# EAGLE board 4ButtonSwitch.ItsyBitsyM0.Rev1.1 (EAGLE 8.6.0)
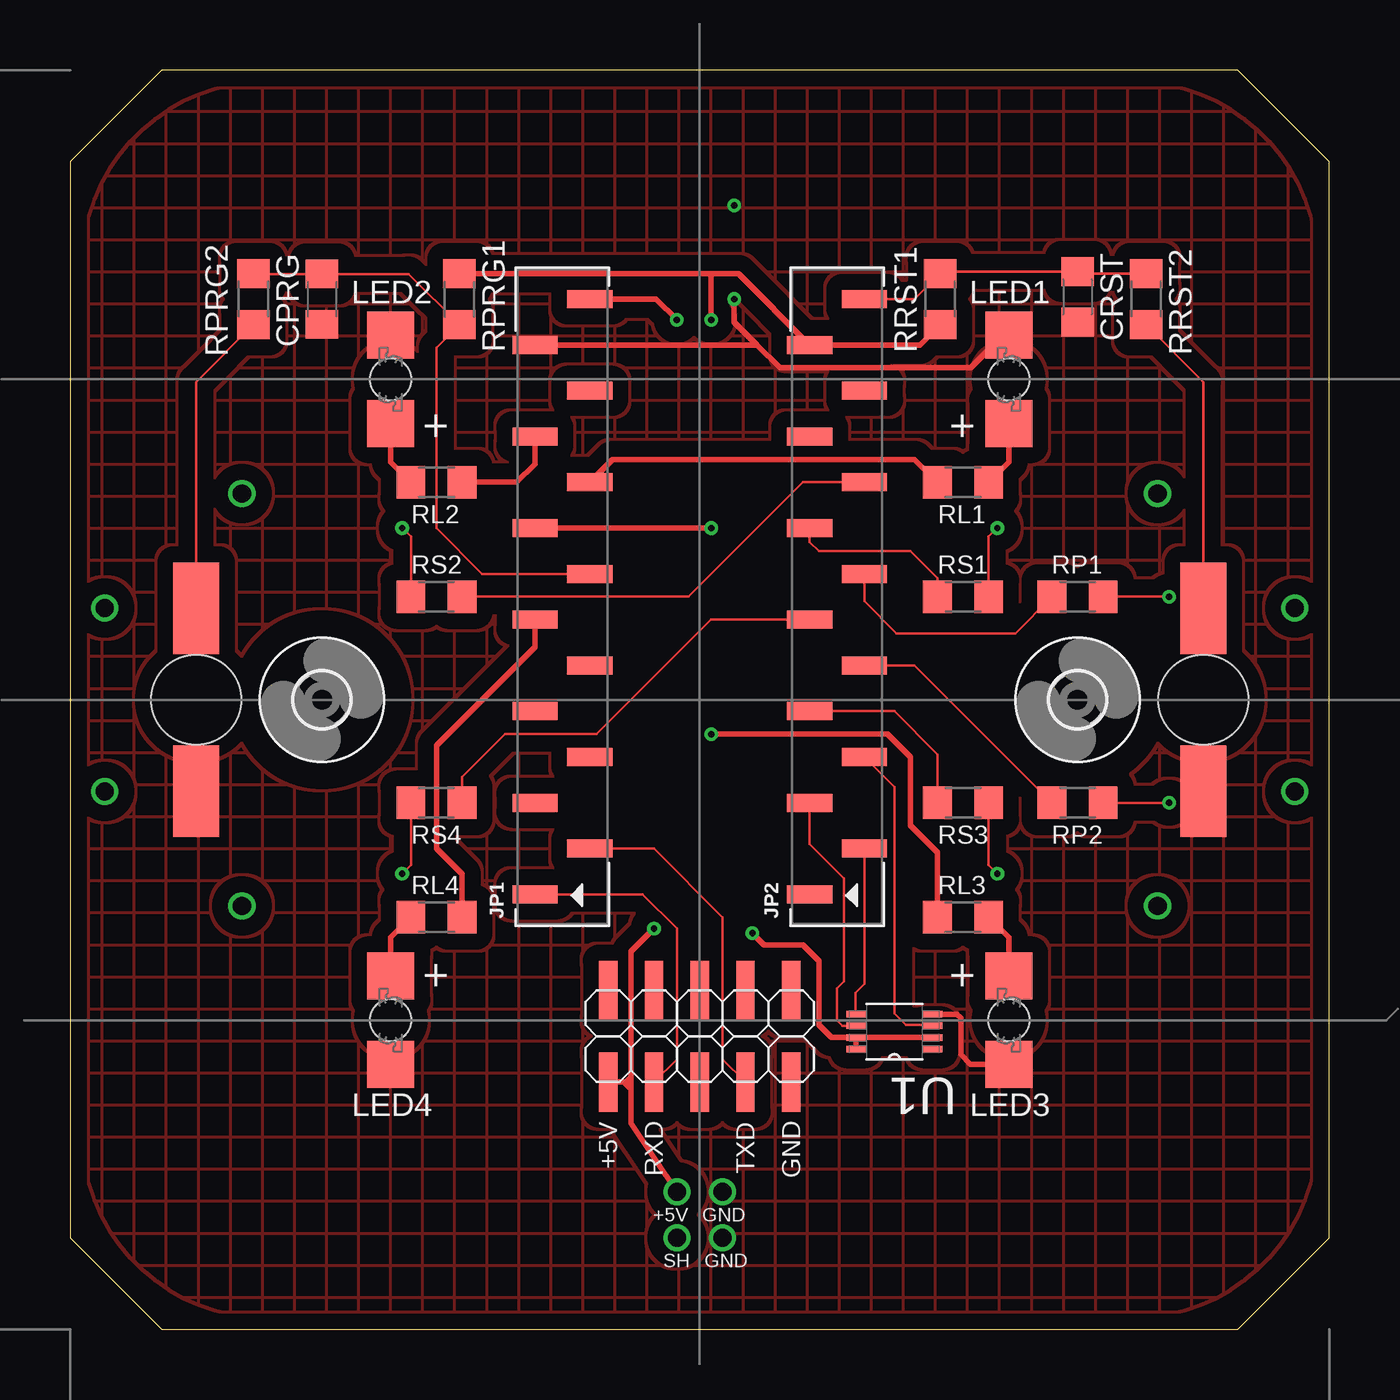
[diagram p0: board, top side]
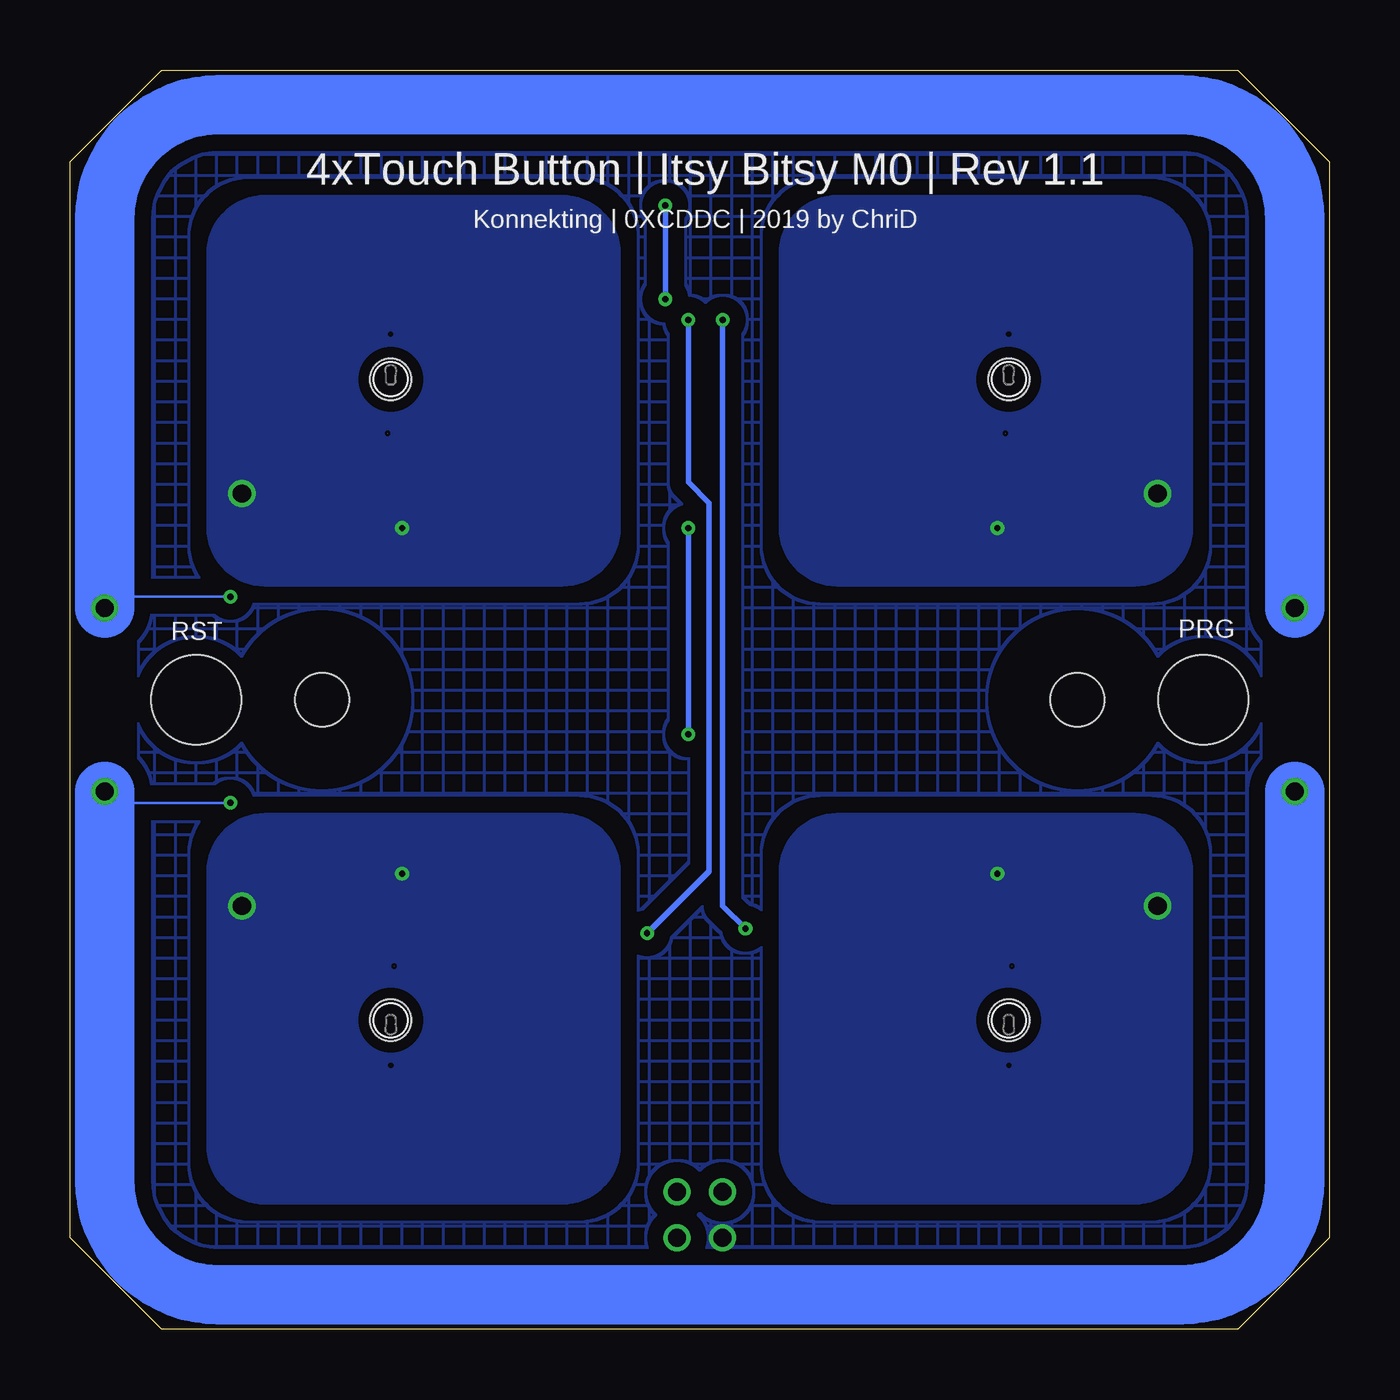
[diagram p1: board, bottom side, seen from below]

Size 69.85 x 69.85 mm. Coordinates in mm from the lower left corner, seen from the top.
Outline: 5.08,69.85 64.77,69.85 69.85,64.77 69.85,5.08 64.77,0 5.08,0 0,5.08 0,64.77 5.08,69.85
Outline: 6.34,69.84 5.08,69.85
Copper layers (1*16): Top 0.035mm / dielectric 1.5mm / Bottom 0.035mm
Design rules "konnektduino": minimum track width 6mil, minimum drill 0.35mm, track to track 6mil, track to pad 6mil, pad to pad 6mil, via to via 6mil, smd to smd 6mil, copper to edge 25mil, drill to drill 6mil, minimum pad ring 10mil, minimum via ring 8mil, stop-mask expansion 1mil, vias tented up to drill 25mil, thermal gap 10mil
Holes 5 mm at 62.87,34.92 6.99,34.92

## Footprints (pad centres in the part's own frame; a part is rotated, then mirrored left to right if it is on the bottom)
C1206 = smd 1.6 x 1.8: 1 -1.4,0; 2 1.4,0
SMD2,54-5,08 = smd 2.54 x 5.08: 1 0,0
1X14_SMT = smd 1 x 2.5: 1 -16.51,1.52; 2 -13.97,-1.52; 3 -11.43,1.52; 4 -8.89,-1.52; 5 -6.35,1.52; 6 -3.81,-1.52; 7 -1.27,1.52; 8 1.27,-1.52; 9 3.81,1.52; 10 6.35,-1.52; 11 8.89,1.52; 12 11.43,-1.52; 13 13.97,1.52; 14 16.51,-1.52
P47F-BOTTOM = smd 2.6 x 2.6: A -2.45,0; C 2.45,0 | hole 2.3: 0,0
R1206 = smd 1.6 x 1.803: 1 -1.422,0; 2 1.422,0
2X05SMD = smd 1.016 x 3.302: 1 -1.27,-3.81; 2 -1.27,1.27; 3 1.27,-3.81; 4 1.27,1.27; 5 3.81,-3.81; 6 3.81,1.27; 7 6.35,-3.81; 8 6.35,1.27; 9 8.89,-3.81; 10 8.89,1.27
SOP65P490X110-8N = smd 1.067 x 0.356: 1 -2.134,0.965; 2 -2.134,0.33; 3 -2.134,-0.33; 4 -2.134,-0.965; 5 2.134,-0.965; 6 2.134,-0.33; 7 2.134,0.33; 8 2.134,0.965
3,0 = hole 3: 0,0

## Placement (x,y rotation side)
CPRG  100nF  [C1206]  13.97,57.15 270 top
CRST  100nF  [C1206]  55.88,57.28 270 top
GND_NRST  0  [SMD2,54-5,08]  6.99,29.84 0 top
GND_PRG  0  [SMD2,54-5,08]  62.87,29.84 0 top
JP1  [1X14_SMT]  27.3,40.64 90 top
JP2  [1X14_SMT]  42.55,40.64 90 top
LED1  LWP4-BOTTOM  [P47F-BOTTOM]  52.07,52.7 90 top
LED2  LWP4-BOTTOM  [P47F-BOTTOM]  17.78,52.7 90 top
LED3  LWP4-BOTTOM  [P47F-BOTTOM]  52.07,17.14 270 top
LED4  LWP4-BOTTOM  [P47F-BOTTOM]  17.78,17.14 270 top
PAD_NRST  0  [SMD2,54-5,08]  62.87,40.01 0 top
PAD_PRG  0  [SMD2,54-5,08]  6.99,40.01 0 top
RL1  330E  [R1206]  49.53,46.99 0 top
RL2  330E  [R1206]  20.32,46.99 180 top
RL3  330E  [R1206]  49.53,22.86 0 top
RL4  330E  [R1206]  20.32,22.86 180 top
RP1  1k  [R1206]  55.88,40.64 180 top
RP2  1k  [R1206]  55.88,29.21 180 top
RPRG1  10k  [R1206]  21.59,57.15 90 top
RPRG2  330E  [R1206]  10.16,57.15 270 top
RRST1  10k  [R1206]  48.26,57.15 270 top
RRST2  330E  [R1206]  59.69,57.15 270 top
RS1  1k  [R1206]  49.53,40.64 180 top
RS2  1k  [R1206]  20.32,40.64 0 top
RS3  1k  [R1206]  49.53,29.21 180 top
RS4  1k  [R1206]  20.32,29.21 0 top
SAM12235-ND  SIEMENS BCU  [2X05SMD]  31.11,17.53 0 top
U1  MAX31723MUA+T  [SOP65P490X110-8N]  45.72,16.51 180 top
U$1  [3,0]  13.97,34.92 0 top
U$2  [3,0]  55.88,34.92 0 top

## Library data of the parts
CPRG CRST = rcl; SPICEPREFIX: C
GND_NRST GND_PRG PAD_NRST PAD_PRG = wirepad
JP1 JP2 = pinhead+
LED1-LED4 = led
RL1-RL4 RP1 RP2 RPRG1 RPRG2 RRST1 RRST2 RS1-RS4 = resistor
SAM12235-ND = pinhead
U1 = MAX31723MUA_T (1); AVAILABILITY: Unavailable; DESCRIPTION: Thermostat Â±2Â°C Digital SMD 8-Pin uMAX T/R; MF: Maxim Integrated; MP: MAX31723MUA+T; PACKAGE: MSOP-8 Maxim Integrated; PRICE: None
U$1 U$2 = holes

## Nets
+3V3: JP2.13 RPRG1.2 RRST1.2 U1.2 U1.7 U1.8
+5V: JP1.14 SAM12235-ND.1
A0: JP2.10 RS2.2
A1: JP2.9 RS1.2
A2: JP2.8 RP1.2
A3: JP2.7 RS4.2
A4: JP2.6 RP2.2
A5: JP2.5 RS3.2
D7: JP1.6
D9: JP1.7 RL4.1
D10: CPRG.1 JP1.8 RPRG1.1 RPRG2.1
D11: JP1.9 RL3.1
D12: JP1.10 RL1.1
D13: JP1.11 RL2.1
GND: CPRG.2 CRST.2 GND_NRST.1 GND_PRG.1 JP1.13 LED1.C LED2.C LED3.C LED4.C SAM12235-ND.9 U1.4
MISO: JP2.2 U1.5
MOSI: JP2.3 U1.6
N$19: LED1.A RL1.2
N$20: LED2.A RL2.2
N$21: LED3.A RL3.2
N$22: LED4.A RL4.2
PRG: PAD_PRG.1 RPRG2.2
RESET: PAD_NRST.1 RRST2.2
RST: CRST.1 JP2.14 RRST1.1 RRST2.1
SCK: JP2.4 U1.3
SCL: JP1.4
SDA: JP1.3
SENS_1: RS1.1
SENS_2: RS2.1
SENS_3: RS3.1
SENS_4: RS4.1
SENS_PROX_1: RP1.1
SENS_PROX_2: RP2.1
USART1_RX: JP1.1 SAM12235-ND.3
USART1_TX: JP1.2 SAM12235-ND.7

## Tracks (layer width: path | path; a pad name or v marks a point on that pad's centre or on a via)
+3V3  (via drill 0.35)
  Top 0.305: 35.56,58.57 37.06,58.57 JP2.13 47.14,54.61 RRST1.2 | 35.56,58.57 RPRG1.2 | U1.8 U1.7 | U1.7 U1.2 | 35.56,58.57 v35.56,56.01 | v37.85,21.97 38.48,21.34 40.64,21.34 41.53,20.45 41.53,16.89 42.24,16.18 U1.7
  Bottom 0.305: v35.56,56.01 35.56,46.99 34.42,45.85 34.42,25.4 v37.85,21.97
+5V  (via drill 0.35, 1)
  Top 0.305: SAM12235-ND.1 30.73,13.72 | 30.73,13.72 30.86,13.72 31.11,13.97 | JP1.14 32.51,57.15 v33.66,56.01 | v33.66,7.62 31.11,11.43 31.11,13.34 | 31.11,13.34 31.11,13.97 | 30.73,13.72 31.11,13.34 | 31.11,13.97 31.11,20.95 v32.38,22.23
  Bottom 0.305: v32.38,22.23 33.66,23.5 v33.66,56.01
A0
  Top 0.152: RS2.2 34.29,40.64 40.64,46.99 JP2.10
A1
  Top 0.152: JP2.9 41.02,43.68 41.53,43.18 46.61,43.18 48.11,41.68 RS1.2
A2
  Top 0.152: JP2.8 44.06,40.39 45.85,38.61 52.43,38.61 RP1.2
A3
  Top 0.152: RS4.2 21.74,30.63 24.13,33.02 29.21,33.02 35.56,39.37 JP2.7
A4
  Top 0.152: JP2.6 46.84,36.83 RP2.2
A5
  Top 0.152: RS3.2 48.11,31.9 45.72,34.29 JP2.5
D9
  Top 0.305: RL4.1 21.74,25.25 20.32,26.67 20.32,32.38 25.79,37.85 JP1.7
D10
  Top 0.152: RPRG2.1 10.18,58.55 CPRG.1 18.77,58.55 RPRG1.1 20.32,54.46 20.32,44.45 22.86,41.91 JP1.8
D11  (via drill 0.35)
  Top 0.305: v35.56,44.45 JP1.9 | v35.56,33.02 45.34,33.02 46.61,31.75 46.61,27.94 48.11,26.44 RL3.1
  Bottom 0.305: v35.56,44.45 v35.56,33.02
D12
  Top 0.305: RL1.1 46.84,48.26 30.09,48.26 JP1.10
D13
  Top 0.305: JP1.11 25.79,48.01 24.77,46.99 RL2.1
GND  (via drill 0.35, 1)
  Top 0.305: 38.1,54.61 39.37,53.34 49.97,53.34 51.27,54.64 51.56,54.64 LED1.C | JP1.13 38.1,54.61 | U1.4 49.2,17.48 49.4,17.27 49.4,15.24 49.95,14.7 LED3.C | 38.1,54.61 36.83,55.88 v36.83,57.15
  Bottom 0.305: v36.83,57.15 v36.83,62.36
  other vias: 36.2,7.62 36.2,5.08
  pour Top (isolate 0.889, rank 6, no thermals, hatched): 0.64,10.79 arc90 10.79,0.64 59.05,0.64 arc90 69.22,10.79 69.22,59.05 arc90 59.05,69.22 10.79,69.22 arc90 0.64,59.05
MISO
  Top 0.152: JP2.2 44.06,19.17 43.56,18.67 43.56,17.5 U1.5
MOSI
  Top 0.152: JP2.3 41.02,26.92 42.93,25.02 42.93,19.3 42.55,18.92 42.55,17.14 42.85,16.84 U1.6
N$19
  Top 0.305: LED1.A 52.07,48.11 RL1.2
N$20
  Top 0.305: LED2.A 17.78,48.11 RL2.2
N$21
  Top 0.305: LED3.A 52.07,21.74 RL3.2
N$22
  Top 0.305: LED4.A 17.78,21.74 RL4.2
PRG
  Top 0.152: PAD_PRG.1 6.99,52.55 RPRG2.2
RESET
  Top 0.152: PAD_NRST.1 62.87,52.55 RRST2.2
RST
  Top 0.152: RRST2.1 55.99,58.57 CRST.1 48.37,58.68 RRST1.1 46.84,57.15 JP2.14
SCK
  Top 0.152: JP2.4 45.72,30.09 45.72,17.53 46.35,16.89 47.8,16.89 U1.3
SENS_1  (via drill 0.35, 1)
  Top 0.152: RS1.1 50.95,43.97 v51.44,44.45
  other vias: 60.33,46.35
  pour Bottom: 39.37,59.69 39.37,44.45 arc90 42.55,41.27 59.05,41.27 arc90 62.23,44.45 62.23,59.69 arc90 59.05,62.87 42.55,62.87 arc90
SENS_2  (via drill 0.35, 1)
  Top 0.152: RS2.1 18.9,43.97 v18.41,44.45
  other vias: 9.53,46.35
  pour Bottom: 10.79,41.27 27.3,41.27 arc90 30.48,44.45 30.48,59.69 arc90 27.3,62.87 10.79,62.87 arc90 7.62,59.69 7.62,44.45 arc90
SENS_3  (via drill 0.35, 1)
  Top 0.152: RS3.1 50.95,25.76 v51.44,25.27
  other vias: 60.33,23.5
  pour Bottom: 59.05,28.57 42.55,28.57 arc90 39.37,25.4 39.37,10.16 arc90 42.55,6.99 59.05,6.99 arc90 62.23,10.16 62.23,25.4 arc90
SENS_4  (via drill 0.35, 1)
  Top 0.152: RS4.1 18.9,25.76 v18.41,25.27
  other vias: 9.53,23.5
  pour Bottom: 7.62,10.16 7.62,25.4 arc-90 10.79,28.57 27.3,28.57 arc-90 30.48,25.4 30.48,10.16 arc-90 27.3,6.99 10.79,6.99 arc-90
SENS_PROX_1  (via drill 0.35, 1)
  Top 0.152: RP1.1 v60.96,40.64
  Bottom 0.152: v67.94,40.01 67.31,40.64 v60.96,40.64
  Bottom 3.302: v1.91,40.01 1.91,61.59 arc-90 8.26,67.94 61.59,67.94 arc-90 67.94,61.59 v67.94,40.01
SENS_PROX_2  (via drill 0.35, 1)
  Top 0.152: RP2.1 v60.96,29.21
  Bottom 0.152: v60.96,29.21 67.31,29.21 v67.94,29.84
  Bottom 3.302: v1.91,29.84 1.91,8.26 arc90 8.26,1.91 61.59,1.91 arc90 67.94,8.26 v67.94,29.84
SHIELD_OR_GND  (via drill 1)
  other vias: 33.66,5.08
  pour Bottom (isolate 0.889, rank 6, no thermals, hatched): 3.81,9.53 arc90 9.53,3.81 60.33,3.81 arc90 66.04,9.53 66.04,60.33 arc90 60.33,66.04 9.53,66.04 arc90 3.81,60.33
USART1_RX
  Top 0.152: JP1.1 31.75,24.13 33.66,22.23 33.66,14.99 SAM12235-ND.3
USART1_TX
  Top 0.152: SAM12235-ND.7 36.2,14.99 36.2,22.86 32.38,26.67 JP1.2

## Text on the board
tNames: + | + | + | + | +5V | RXD | TXD | GND | +5V | GND | SH | GND
bNames: 4xTouch Button | Itsy Bitsy M0 | Rev 1.1 | Konnekting | 0XCDDC | 2019 by ChriD | PRG | RST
